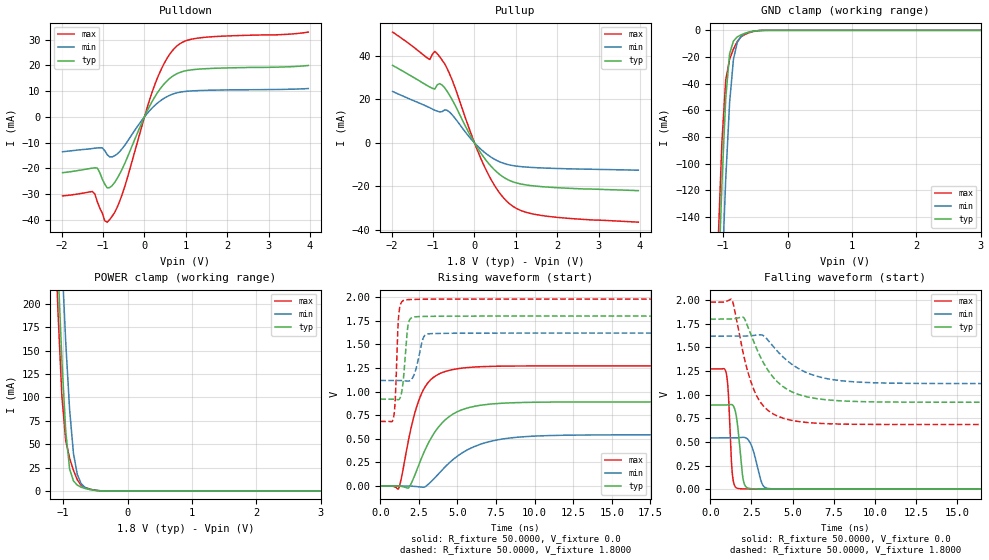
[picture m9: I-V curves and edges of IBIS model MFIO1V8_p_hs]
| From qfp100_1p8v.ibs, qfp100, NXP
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[Model] MFIO1V8_p_hs
|   Model MFIO1V8_p_hs
| This model was characterised for following simulation conditions:
| External (pad) voltage:
|   - Typ: 1.8V,   - Min: 1.62V,   - Max: 1.98V
| Library cells for typ/min/max conditions are connected as defined below:
|  IO - External Pad
|  A - Core Input
|  EN - Output Buffer Enable
|  BOOST - vdde
|  EHS - vdd
|  ENZI - vdd
|  EPD - gnd
|  EPUN - vdd
|  ZI - NC
|  ZIF - NC
|  gnd - gnd
|  gnde - gnde
|  vdd - vdd
|  vdde - vdde
| All other pins connected to ground
Model_type I/O
Polarity   Non-Inverting
Enable   Active-Low
Vinl =   0.5400V
Vinh =   1.2600V
Vmeas =  0.9000V
Cref =   0.0F
Rref =   100.0000
Vref =   0.0V
C_comp   1.6238pF   1.5412pF   1.6971pF
|C_comp_pullup   0.8047pF   0.8356pF   0.7616pF
|C_comp_pulldown   0.6044pF   0.6428pF   0.5687pF
[Model Spec]
| variable   typ   min   max
Vinh   0.5400V   0.4860V   0.5940V
Vinl   1.2600V   1.1340V   1.3860V
Vmeas   0.9000V   0.8100V   0.9900V
[Temperature Range]   25.0000   0.1250k   -40.0000
[Voltage Range]   1.8000V   1.6200V   1.9800V
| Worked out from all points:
|   slope of the pulldown table from 0 to 0.27 V, typ, clamps not added: 32.6 ohm
|   slope of the pullup table from 0 to 0.27 V, typ, clamps not added: 34.8 ohm
|   GND clamp passes 1 mA (typ) near -0.56 V on its own axis
|   POWER clamp passes 1 mA (typ) near -0.54 V on its own axis
|   rising waveform, R_fixture 50.0000, V_fixture 0.0: 20-80 % time 1.9ns typ, 2.68ns min, 1.22ns max; typ from 0 V to 0.89 V
|   rising waveform, R_fixture 50.0000, V_fixture 1.8000: 20-80 % time 264ps typ, 419ps min, 177ps max; typ from 0.92 V to 1.8 V
|   falling waveform, R_fixture 50.0000, V_fixture 0.0: 20-80 % time 304ps typ, 487ps min, 202ps max; typ from 0.89 V to 0 V
|   falling waveform, R_fixture 50.0000, V_fixture 1.8000: 20-80 % time 1.84ns typ, 2.29ns min, 1.29ns max; typ from 1.8 V to 0.92 V
[Pulldown]
|Voltage   I(typ)   I(min)   I(max)
-1.98V    -21.74mA   -13.58mA   -30.76mA
-1.26V    -19.96mA   -12.33mA   -29.04mA
-1.14V    -19.96mA   -12.1mA    -33mA
-960mV    -26.19mA   -13.15mA   -40.44mA
-840mV    -27.51mA   -15.58mA   -39.92mA
-540mV    -20.34mA   -12.41mA   -30.2mA
60mV      2.086mA    1.197mA    3.341mA
300mV     9.043mA    5.145mA    14.58mA
540mV     13.88mA    7.813mA    22.59mA
840mV     17.16mA    9.517mA    28.23mA
1.44V     18.67mA    10.27mA    30.87mA
3.96V     19.95mA    10.98mA    32.93mA
[Pullup]
|Voltage   I(typ)   I(min)   I(max)
-1.98V    35.7mA     23.68mA    51.03mA
-1.08V    25.71mA    16.17mA    38.42mA
-960mV    24.81mA    15.04mA    42.18mA
-840mV    27.29mA    14.27mA    39.65mA
-720mV    25.36mA    15.21mA    36.42mA
-540mV    19.88mA    12.94mA    28.95mA
-60mV     2.002mA    1.263mA    3.041mA
240mV     -7.02mA    -4.333mA   -10.88mA
600mV     -14.41mA   -8.644mA   -22.88mA
900mV     -17.74mA   -10.36mA   -28.83mA
1.74V     -20.33mA   -11.62mA   -33.75mA
3.96V     -22mA      -12.58mA   -36.53mA
[GND_clamp]
|Voltage   I(typ)   I(min)   I(max)
-1.98V    -1.781A    -1.801A    -1.77A
-1.08V    -200.1mA   -270.2mA   -162.2mA
-1.02V    -116mA     -186.2mA   -84.48mA
-960mV    -51.25mA   -111.8mA   -37.35mA
-900mV    -17.64mA   -54.43mA   -21.68mA
-840mV    -8.011mA   -21.69mA   -14.07mA
-780mV    -4.915mA   -8.957mA   -8.303mA
-720mV    -3.329mA   -4.435mA   -4.743mA
-600mV    -1.395mA   -1.331mA   -1.886mA
-480mV    -322.5uA   -340.7uA   -414uA
-360mV    -20uA      -33.74uA   -21.95uA
3.96V     0A         0A         0A
[POWER_clamp]
|Voltage   I(typ)   I(min)   I(max)
-1.98V    2.119A     2.147A     2.105A
-1.14V    349.2mA    449.9mA    300.5mA
-1.08V    239.1mA    345.9mA    191.2mA
-1.02V    140.3mA    247.7mA    101.6mA
-960mV    64.04mA    159.3mA    53.83mA
-900mV    23.55mA    87.2mA     35.06mA
-840mV    10.74mA    40.16mA    22.02mA
-780mV    6.173mA    17.47mA    11.87mA
-720mV    3.968mA    7.718mA    5.953mA
-600mV    1.695mA    1.811mA    2.312mA
-360mV    25.02uA    62.74uA    19.06uA
3.96V     0A         0A         0A
[Ramp]
| variable   typ   min   max
dV/dt_r  0.5342/1.9018n   0.3254/2.6766n   0.7634/1.2229n
dV/dt_f  0.5279/1.8432n   0.3012/2.2950n   0.7772/1.2878n
R_load = 50.0000
[Rising Waveform]
R_fixture= 50.0000
V_fixture= 0.0
V_fixture_min= 0.0
V_fixture_max= 0.0
|time   V(typ)   V(min)   V(max)
0s        1.152nV    106.1nV    55.38pV
1.185ns   -403.2uV   61.31uV    -28.45mV
1.827ns   -20.54mV   -119.8uV   484.8mV
2.193ns   96.9mV     -3.411mV   747.4mV
3.078ns   443mV      14.04mV    1.092V
4.202ns   700.3mV    202.8mV    1.213V
5.785ns   832.9mV    394.6mV    1.257V
8.37ns    880.6mV    508.2mV    1.27V
12.97ns   890.1mV    540.1mV    1.272V
100ns     890.4mV    542.4mV    1.272V
[Rising Waveform]
R_fixture= 50.0000
V_fixture= 1.8000
V_fixture_min= 1.6200
V_fixture_max= 1.9800
|time   V(typ)   V(min)   V(max)
0s        920.2mV    1.118V     684.7mV
851.4ps   920.4mV    1.118V     717.1mV
968.1ps   918.1mV    1.118V     907.6mV
1.215ns   917.2mV    1.119V     1.843V
1.467ns   1.085V     1.116V     1.962V
1.737ns   1.622V     1.111V     1.973V
2.222ns   1.791V     1.192V     1.977V
2.82ns    1.796V     1.581V     1.978V
3.428ns   1.798V     1.615V     1.979V
100ns     1.8V       1.62V      1.98V
[Falling Waveform]
R_fixture= 50.0000
V_fixture= 0.0
V_fixture_min= 0.0
V_fixture_max= 0.0
|time   V(typ)   V(min)   V(max)
0s        890.4mV    542.4mV    1.272V
965.1ps   890.7mV    542.4mV    1.231V
1.093ns   893.1mV    542.3mV    1.025V
1.359ns   889.9mV    542.1mV    130.6mV
1.581ns   770.6mV    543.3mV    14.25mV
1.813ns   401mV      546.8mV    4.559mV
2.153ns   27.07mV    543.9mV    2.301mV
3.169ns   1.789mV    48.93mV    729.1uV
3.838ns   975.3uV    3.271mV    392uV
100ns     11.14nV    121.7nV    6.012nV
[Falling Waveform]
R_fixture= 50.0000
V_fixture= 1.8000
V_fixture_min= 1.6200
V_fixture_max= 1.9800
|time   V(typ)   V(min)   V(max)
0s        1.8V       1.62V      1.98V
1.324ns   1.801V     1.62V      2.006V
1.983ns   1.821V     1.62V      1.45V
2.289ns   1.717V     1.622V     1.237V
2.739ns   1.518V     1.629V     1.016V
3.215ns   1.341V     1.627V     882.6mV
4.41ns    1.087V     1.401V     751.8mV
6.133ns   968mV      1.214V     701.9mV
12.93ns   920.6mV    1.119V     684.7mV
100ns     920.2mV    1.118V     684.7mV
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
